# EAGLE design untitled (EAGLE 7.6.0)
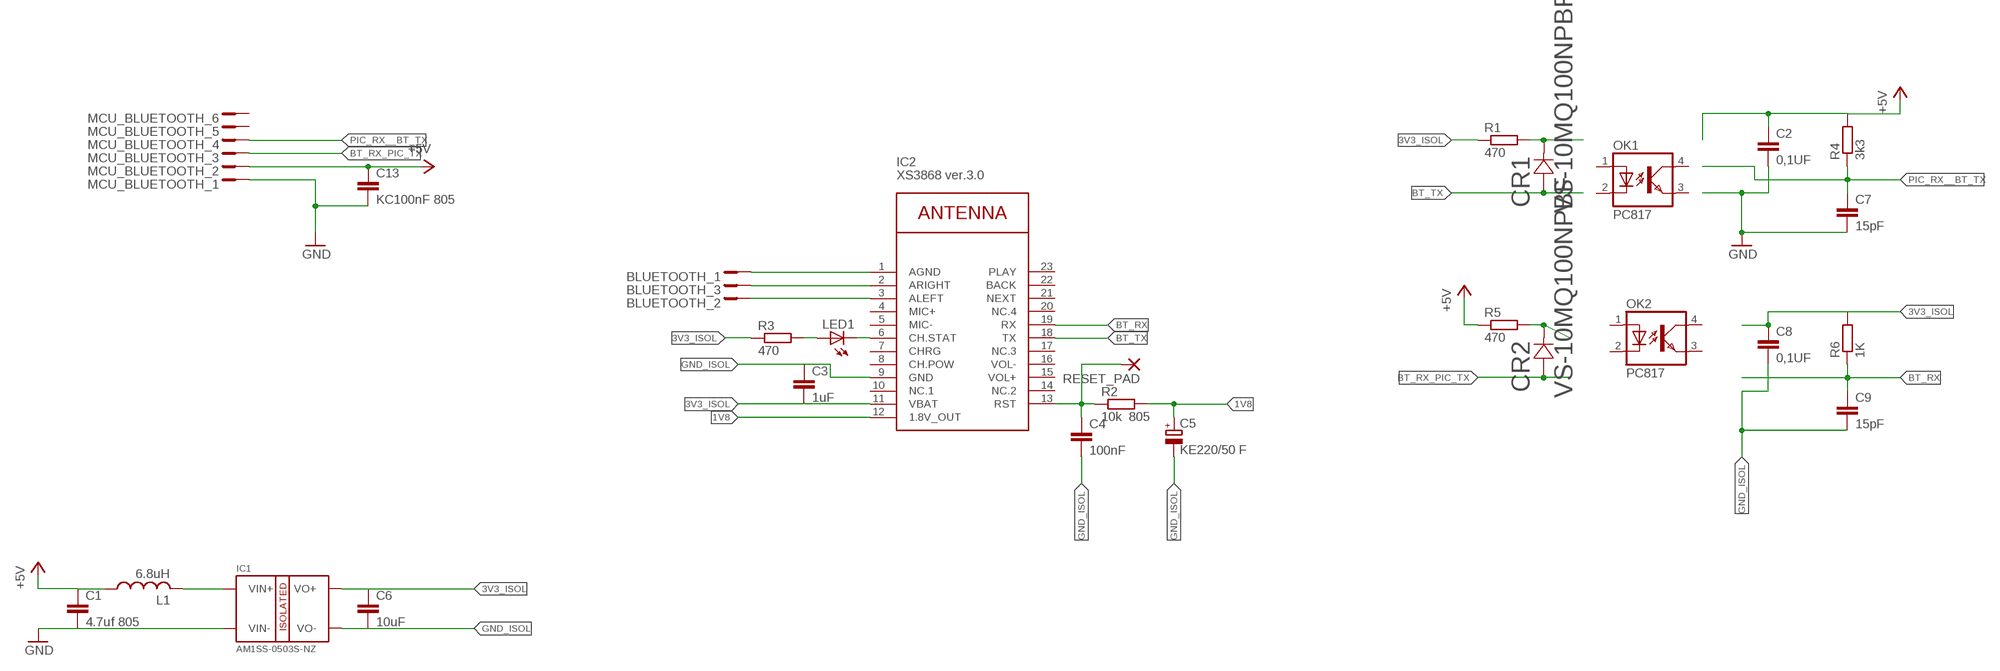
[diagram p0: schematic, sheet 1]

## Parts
BLUETOOTH  JST_3_PIN_B3B-PH-KS  [B3B-PH-KS]
C1  4.7uf 805  C-EUC0805  [C0805]
C2  0,1UF  C-EUC0805  [C0805]
C3  1uF  C-EUC0805  [C0805]
C4  100nF  C-EUC0805  [C0805]
C5  KE220/50 F  CPOL-EUG  [PANASONIC_G]
C6  10uF  C-EUC0805  [C0805]
C7  15pF  C-EUC0805  [C0805]
C8  0,1UF  C-EUC0805  [C0805]
C9  15pF  C-EUC0805  [C0805]
C13  KC100nF 805  C-EUC0805  [C0805]
CR1  VS-10MQ100NPBF  [DIODE_SMA]
CR2  VS-10MQ100NPBF  [DIODE_SMA]
IC1  AM1SS-0503S-NZ  [SIP4]
IC2  XS3868 ver.3.0  WIRELESS-BLUETOOTH-XS3868  [WIRELESS-BLUETOOTH-XS3868]
L1  6.8uH  L-US0204/5  [0204/5]
LED1  LEDSMART-LED  [SMART-LED]
MCU_BLUETOOTH  JST_6_PIN_B6B-PH-KS  [B6B-PH-KS]
OK1  PC817  [DIL04]
OK2  PC817  [DIL04]
R1  470  R-EU_M0805  [M0805]
R2  10k 805  R-EU_M0805  [M0805]
R3  470  R-EU_M0805  [M0805]
R4  3k3  R-EU_M0805  [M0805]
R5  470  R-EU_M0805  [M0805]
R6  1K  R-EU_M0805  [M0805]
RESET_PAD  SMD2  [SMD1,27-2,54]

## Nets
1V8: C5.+ IC2.12(1.8V_OUT) R2.2
3V3_ISOL: C3.2 C6.1 C8.1 IC1.P$3(VO+) IC2.11(VBAT) R1.1 R3.1 R6.2
+5V: C1.1 C2.1 C13.1 L1.1 MCU_BLUETOOTH.P$2 R4.2 R5.1
AGND: BLUETOOTH.P$1 IC2.1(AGND)
BT_LED: IC2.6(CH.STAT) LED1.B(C)
BT_RX: C9.1 IC2.19(RX) R6.1
BT_RX_PIC_TX: CR2.2 MCU_BLUETOOTH.P$3
BT_TX: CR1.2 IC2.18(TX)
BTOUT_LEFT: BLUETOOTH.P$2 IC2.3(ALEFT)
BTOUT_RIGHT: BLUETOOTH.P$3 IC2.2(ARIGHT)
GND: C1.2 C2.2 C7.2 C13.2 IC1.P$2(VIN-) MCU_BLUETOOTH.P$1
GND_ISOL: C3.1 C4.2 C5.- C6.2 C8.2 C9.2 IC1.P$4(VO-) IC2.9(GND)
N$1: IC1.P$1(VIN+) L1.2
N$2: CR1.1 R1.2
N$3: CR2.1 R5.2
N$5: LED1.A R3.2
PIC_RX__BT_TX: C7.1 MCU_BLUETOOTH.P$4 R4.1
RST: C4.1 IC2.13(RST) R2.1 RESET_PAD.1(P)
Unconnected: IC2.4(MIC+) IC2.5(MIC-) IC2.7(CHRG) IC2.8(CH.POW) IC2.10(NC.1) IC2.14(NC.2) IC2.15(VOL+) IC2.16(VOL-) IC2.17(NC.3) IC2.20(NC.4) IC2.21(NEXT) IC2.22(BACK) IC2.23(PLAY) MCU_BLUETOOTH.P$5 MCU_BLUETOOTH.P$6 OK1.1(A) OK1.2(C) OK1.3(EMIT) OK1.4(COL) OK2.1(A) OK2.2(C) OK2.3(EMIT) OK2.4(COL)

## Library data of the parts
BLUETOOTH = conn-JST:JST_3_PIN_
C1 C13 = rcl:C-EU: CAPACITOR, European symbol
C2-C4 C6-C9 = resistor:C-EU: CAPACITOR, European symbol
C5 = rcl:CPOL-EU: POLARIZED CAPACITOR, European symbol
CR1 CR2 = untitled:VS-10MQ100NPBF; MANUFACTURER_PART_NUMBER: VS10MQ100NPBF; VENDOR: Vishay
IC1 = DC-DC_converter:AM1SS
IC2 = diy-modules:WIRELESS-BLUETOOTH-XS3868: Bluetooth Stereo Audio Module based on OVC3860 chip More details available here: http://artofcircuits.com/product/bluetooth-2-0-edr-stereo-audio-ovc3860-module-model-xs-3868 Click here to find device on ebay.com
L1 = rcl:L-US: INDUCTOR, American symbol
LED1 = led:LED: LED
MCU_BLUETOOTH = conn-JST:JST_6_PIN_
OK1 OK2 = optocoupler:PC817: SHARP OPTO COUPLER; MPN: PC817X4J000F; OC_FARNELL: 9707727; OC_NEWARK: 97K7059
R1-R6 = rcl:R-EU_: RESISTOR, European symbol
RESET_PAD = wirepad:SMD2: SMD PAD

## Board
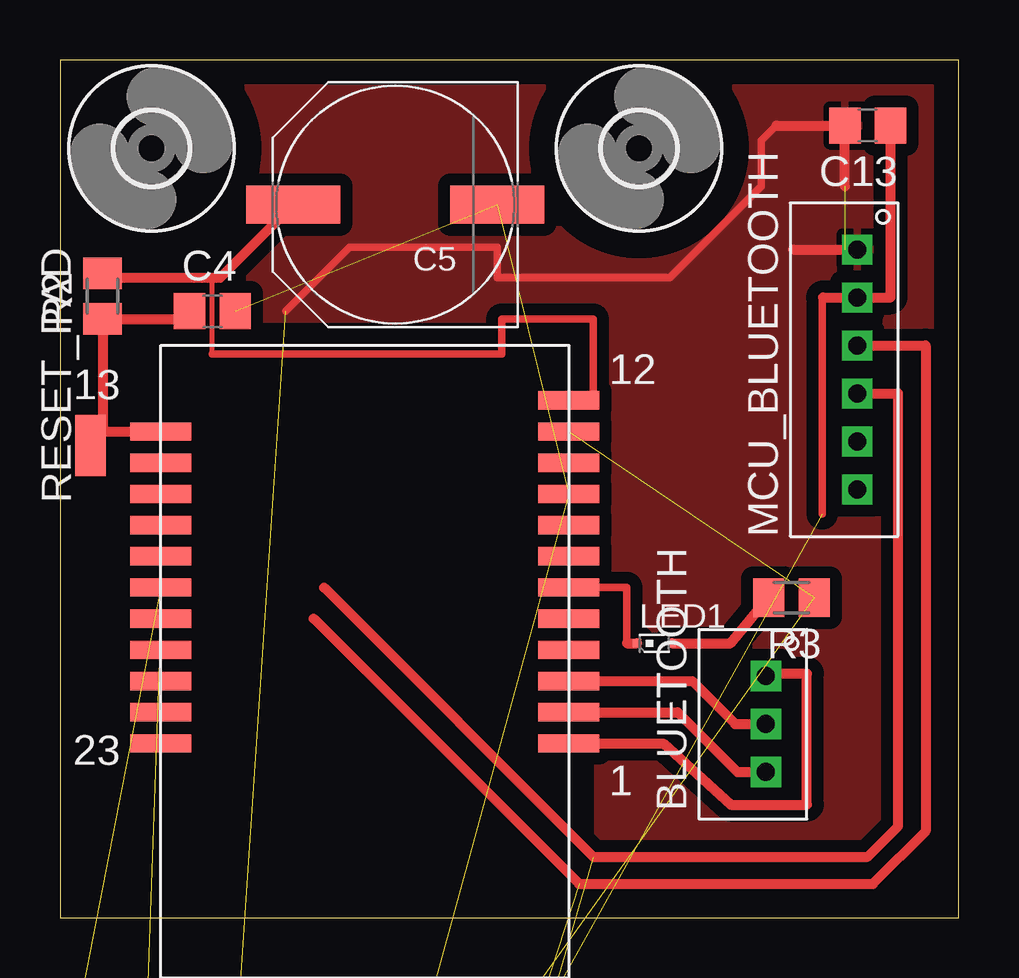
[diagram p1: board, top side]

Size 37.45 x 35.75 mm. Coordinates in mm from the lower left corner, seen from the top.
Outline: 0,0 37.45,0 37.45,35.75 0,35.75 0,0
Copper layers (1*16): Top 0.035mm / dielectric 1.5mm / Bottom 0.035mm
Design rules "default": minimum track width 10mil, minimum drill 24mil, track to track 8mil, track to pad 8mil, pad to pad 8mil, via to via 8mil, smd to smd 8mil, copper to edge 40mil, drill to drill 8mil, minimum pad ring 10mil, minimum via ring 8mil, stop-mask expansion 4mil, vias tented up to drill 0mil, thermal gap 10mil
tRestrict: area 3.8,-7 to 21.6,24.1

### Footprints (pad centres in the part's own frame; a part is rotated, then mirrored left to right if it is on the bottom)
B3B-PH-KS = drill 0.75 pad 1.2 square: P$1 -2,1.7; P$2 -4,1.7; P$3 -6,1.7
C0805 = smd 1.3 x 1.5: 1 -0.95,0; 2 0.95,0
PANASONIC_G = smd 3.9 x 1.6: + 4.25,0; - -4.25,0
DIODE_SMA = smd 2.184 x 1.575: 1 -1.702,0; 2 1.702,0
SIP4 = drill 0.6 square: P$1 -0.415,-2.91; P$2 2.035,-2.91; P$3 4.485,-2.91; P$4 6.935,-2.91
WIRELESS-BLUETOOTH-XS3868 = smd 2.54 x 0.762: 1 -8.5,0.995; 2 -8.5,-0.305; 3 -8.5,-1.605; 4 -8.5,-2.905; 5 -8.5,-4.205; 6 -8.5,-5.505; 7 -8.5,-6.805; 8 -8.5,-8.105; 9 -8.5,-9.405; 10 -8.5,-10.705; 11 -8.5,-12.005; 12 -8.5,-13.305; 13 8.5,-12.005; 14 8.5,-10.705; 15 8.5,-9.405; 16 8.5,-8.105; 17 8.5,-6.805; 18 8.5,-5.505; 19 8.5,-4.205; 20 8.5,-2.905; 21 8.5,-1.605; 22 8.5,-0.305; 23 8.5,0.995
0204/5 = drill 0.813 octagon: 1 -2.54,0; 2 2.54,0
SMART-LED = smd 0.35 x 0.35: A 0,0.725; B 0,-0.725
B6B-PH-KS = drill 0.75 pad 1.2 square: P$1 -2,1.7; P$2 -4,1.7; P$3 -6,1.7; P$4 -8,1.7; P$5 -10,1.7; P$6 -12,1.7
DIL04 = drill 0.813 offset: 1 -1.27,-3.81; 2 1.27,-3.81; 3 1.27,3.81; 4 -1.27,3.81
M0805 = smd 1.3 x 1.6: 1 -0.95,0; 2 0.95,0
SMD1,27-2,54 = smd 1.27 x 2.54: 1 0,0
3,0 = hole 3: 0,0

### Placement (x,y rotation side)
BLUETOOTH  31.12,12.06 90 top
C1  not placed on the board
C2  not placed on the board
C3  not placed on the board
C4  6.35,25.27 0 top
C5  13.97,29.72 180 top
C6  not placed on the board
C7  not placed on the board
C8  not placed on the board
C9  not placed on the board
C13  33.66,33.02 180 top
CR1  not placed on the board
CR2  not placed on the board
IC1  not placed on the board
IC2  12.7,8.25 180 top
L1  not placed on the board
LED1  24.77,11.43 270 top
MCU_BLUETOOTH  34.93,29.84 90 top
OK1  not placed on the board
OK2  not placed on the board
R1  not placed on the board
R2  1.78,25.91 90 top
R3  30.48,13.34 180 top
R4  not placed on the board
R5  not placed on the board
R6  not placed on the board
RESET_PAD  1.27,19.68 0 top
U$2  [3,0]  3.81,32.07 0 top
U$3  [3,0]  24.13,32.07 0 top

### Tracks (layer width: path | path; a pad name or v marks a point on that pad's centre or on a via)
1V8
  Top 0.203: 6.35,23.49 6.35,26.67
  Top 0.305: IC2.12 22.23,21.56 22.23,24.96 18.41,24.96 18.41,23.49 6.35,23.49
  Top 0.406: R2.2 1.78,26.67 6.35,26.67 6.67,26.67 C5.+
3V3_ISOL  (7 unrouted)
+5V  (5 unrouted)
  Top 0.305: 31.75,16.83 31.75,25.84 31.8,25.84
  Top 0.406: C13.1 34.61,25.84 MCU_BLUETOOTH.P$2 31.8,25.84
AGND
  Top 0.406: IC2.1 25.12,7.26 27.94,4.7 31.12,4.7 31.12,10.16 29.51,10.16 BLUETOOTH.P$1
BT_LED
  Top 0.305: IC2.6 23.62,13.76 23.62,11.43
  Top 0.406: 23.62,11.43 LED1.B
BT_RX  (2 unrouted)
BT_RX_PIC_TX  (1 unrouted)
  Top 0.406: MCU_BLUETOOTH.P$3 36.07,23.84 36.07,3.6 33.87,1.4 21.63,1.4 10.57,12.46
BT_TX  (1 unrouted)
BTOUT_LEFT
  Top 0.406: BLUETOOTH.P$2 28.13,8.06 26.34,9.86 IC2.3
BTOUT_RIGHT
  Top 0.406: IC2.2 25.73,8.56 28.23,6.06 BLUETOOTH.P$3
GND  (5 unrouted)
  Top 0.305: 32.39,33.02 C13.2 | 29.84,33.02 29.21,32.38 29.21,30.48 25.4,26.67 18.22,26.67 18.22,27.94 12.06,27.94 9.4,25.27 | 32.7,27.84 MCU_BLUETOOTH.P$1
  Top 0.406: 32.71,30.48 C13.2 29.84,33.02 | 30.54,27.84 MCU_BLUETOOTH.P$1
  pour Top (isolate 0.508): -1.9,36.83 38.73,36.83 38.73,-1.27 -1.9,-1.27
GND_ISOL  (7 unrouted)
N$1  (1 unrouted)
N$2  (1 unrouted)
N$3  (1 unrouted)
N$5
  Top 0.305: 29.53,12.7 R3.2
  Top 0.406: LED1.A 27.94,11.43 R3.2
PIC_RX__BT_TX  (2 unrouted)
  Top 0.406: 11.01,13.76 22.23,2.54 33.66,2.54 34.93,3.81 34.93,21.84 MCU_BLUETOOTH.P$4
RST
  Top 0.305: C4.1 5.4,24.96 | RESET_PAD.1 1.85,20.26
  Top 0.406: C4.1 5.08,24.96 R2.1 1.78,20.26 1.85,20.26 IC2.13

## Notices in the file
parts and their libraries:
diy-modules: Released under the Creative Commons Attribution 4.0 International License: http://creativecommons.org/licenses/by/4.0
